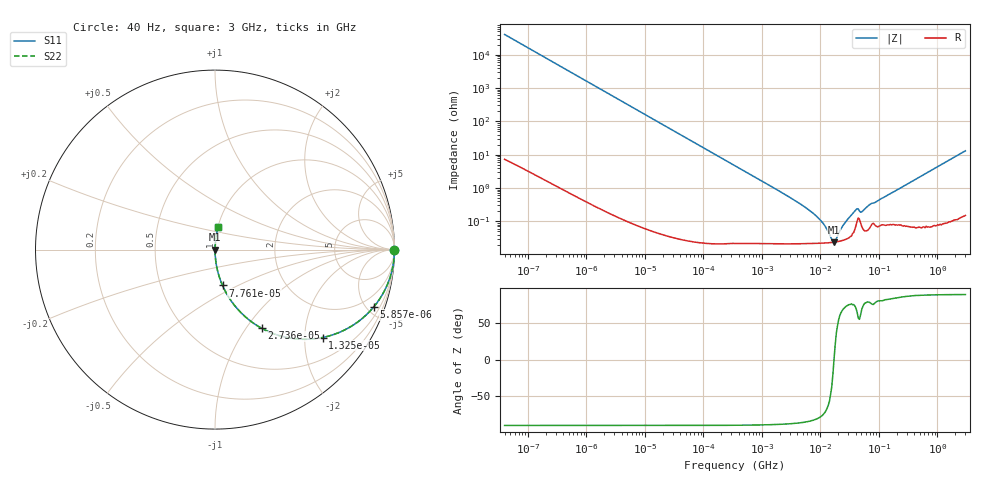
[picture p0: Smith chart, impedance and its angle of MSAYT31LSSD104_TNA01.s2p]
! MSAYT31LSSD104_TNA01  S-PARAMETER MODEL  ( General Type )
! Model Generated by TAIYO YUDEN Corporation (http://www.ty-top.com)
! Version 2.0
! TAIYO YUDEN Control No. 031016
! Copyright(c) 2003 TAIYO YUDEN CO.,LTD. All Rights Reserved.
! Product Description (link to TY-COMPAS)
! https://ds.yuden.co.jp/TYCOMPAS/or/detail?pn=MSAYT31LSSD104KTNA01&u=M
! Products Name : Multilayer Ceramic Capacitors
! Characteristics :
!  Capacitance : 0.1 uF , Rated Voltage : 25V
!  Case Size : 3.2 x 1.6 / 0.126 x 0.063 [mm/inch] , Thickness : 1.6 / 0.063 [mm/inch]
!  (Conditions: Temperature = 25 degC , DC Bias Current/Voltage = 0A / 0V)
! External Node Assignments :
!  1  o---| |---o  2
! GND o---------o GND
! Frequency Range : 40Hz  -  3GHz  [ 401 STEP ]
# MHz S RI R 50
! Freq[MHz].  S11 Real  S11 Imag  S21 Real  S21 Imag  S12 Real  S12 Imag  S22 Real  S22 Imag
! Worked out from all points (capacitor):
!   401 points, 40 Hz to 3 GHz, reference 50 ohm
!   read as one part in series: C = 98.3 nF near 44 Hz
!   lowest |Z| = 23.6 mohm at 17.09 MHz (marker M1)
!   series resonance near 17.04 MHz, so ESL is about 890 pH
!   S11 on the Smith chart (normalised r, x): 40 Hz: open; 5.857 kHz: 1.00, -5.53; 13.25 kHz: 1.00, -2.44; 27.36 kHz: 1.00, -1.18; 77.61 kHz: 1.00, -0.42; 3 GHz: 1.00, +0.26
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4e-05  1 -0.00247  6.55e-06 0.00247  6.55e-06 0.00247  1 -0.00247
0.000834  0.9973 -0.0514  0.00266 0.0514  0.00266 0.0514  0.9973 -0.0514
0.002366  0.9791 -0.1431  0.0209 0.1431  0.0209 0.1431  0.9791 -0.1431
0.005857  0.8842 -0.3198  0.1158 0.3198  0.1158 0.3198  0.8842 -0.3198
0.013246  0.599 -0.4899  0.401 0.4899  0.401 0.4899  0.599 -0.4899
0.017386  0.4645 -0.4985  0.5355 0.4985  0.5355 0.4985  0.4645 -0.4985
0.027358  0.2595 -0.4381  0.7405 0.4381  0.7405 0.4381  0.2595 -0.4381
0.045045  0.1146 -0.3182  0.8854 0.3182  0.8854 0.3182  0.1146 -0.3182
0.077606  0.0419 -0.1998  0.9581 0.1998  0.9581 0.1998  0.0419 -0.1998
0.362475  0.0022 -0.0445  0.9978 0.0445  0.9978 0.0445  0.0022 -0.0445
2.916825  0.00024 -0.00539  0.9998 0.00539  0.9998 0.00539  0.00024 -0.00539
7.222098  0.00022 -0.00183  0.9998 0.00183  0.9998 0.00183  0.00022 -0.00183
10.86056  0.000222 -0.000889  0.9998 0.000889  0.9998 0.000889  0.000222 -0.000889
15.60822  0.000232 -0.000174  0.9998 0.000174  0.9998 0.000174  0.000232 -0.000174
17.08948  0.000236 6.35e-06  0.9998 -6.35e-06  0.9998 -6.35e-06  0.000236 6.35e-06
18.71131  0.000242 0.000183  0.9998 -0.000183  0.9998 -0.000183  0.000242 0.000183
25.69909  0.000279 0.000814  0.9997 -0.000814  0.9997 -0.000814  0.000279 0.000814
38.64618  0.000573 0.00196  0.9994 -0.00196  0.9994 -0.00196  0.000573 0.00196
53.07868  0.000601 0.00198  0.9994 -0.00198  0.9994 -0.00198  0.000601 0.00198
69.67004  0.000648 0.00312  0.9994 -0.00312  0.9994 -0.00312  0.000648 0.00312
150.5692  0.000826 0.00647  0.9992 -0.00647  0.9992 -0.00647  0.000826 0.00647
3000  0.0182 0.1282  0.9818 -0.1282  0.9818 -0.1282  0.0182 0.1282
